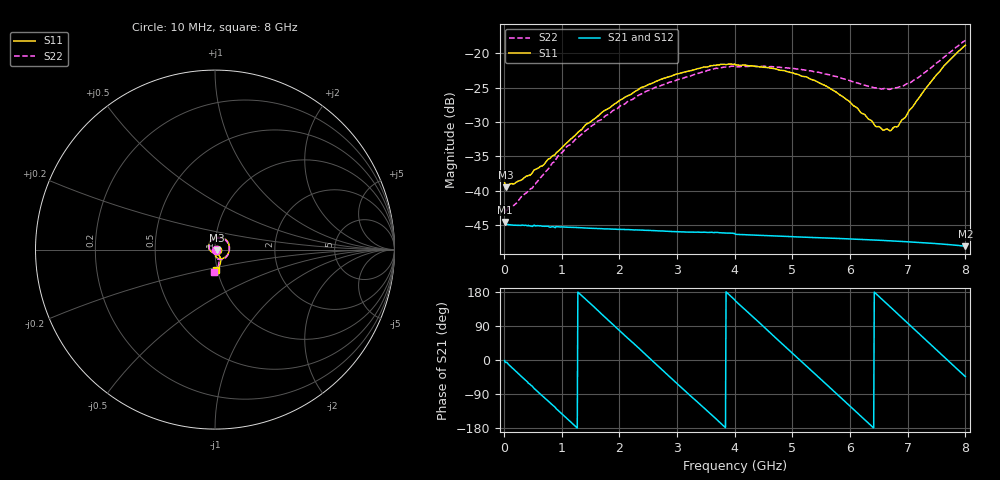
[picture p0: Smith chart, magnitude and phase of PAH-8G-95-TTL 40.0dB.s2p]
! MTS Systemtechnik GmbH
! S-Parameters
! Model: PAH-8G/95-TTL
! Attenuation Step: 40.0dB
! Rohde & Schwarz ZVB8 2Ports - Version 4.11 - 1145.1010k08 SN: 100119
! S2P File Measurements:
! S11 S21 S12 S22
# HZ  S  DB  R  50.00
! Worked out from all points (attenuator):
!   800 points, 10 MHz to 8 GHz, reference 50 ohm
!   highest |S21| = -44.56 dB at 10 MHz (marker M1); lowest = -48.1 dB at 8 GHz (marker M2)
!   lowest |S11| = -39.5 dB at 30 MHz (marker M3), VSWR 1.02, Z = 51.1 - j0.174 ohm
!   |S11| at or under -10 dB: start of sweep to end of sweep
!   |S22| runs from -43.3 to -18.1 dB; largest |S21 - S12| = 8.6e-05
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1e7  -38.85 -11.4  -44.56 -1.2  -44.46 -1.1  -42.43 -16.6
3e7  -39.54 -9.3  -44.97 -6.4  -44.99 -6.4  -43.26 -12.4
1.9e8  -38.94 -28.7  -45.04 -27.6  -45.04 -27.5  -42.01 -34.6
4.5e8  -37.79 -65.9  -45.16 -64.1  -45.17 -63.9  -39.81 -73.9
9.6e8  -34.11 -130.1  -45.29 -135.9  -45.29 -136.1  -34.76 -135.6
1.35e9  -31.06 -169.3  -45.42 169.3  -45.44 169.2  -31.75 -169.4
1.71e9  -28.52 162.2  -45.57 118.7  -45.59 119.1  -29.51 163.7
2.01e9  -26.83 140.2  -45.64 76.4  -45.67 76.6  -27.69 142.7
2.38e9  -24.97 116.1  -45.74 25.0  -45.75 25.0  -25.92 120.3
2.68e9  -23.92 97.5  -45.87 -17.3  -45.85 -17.0  -24.83 102.8
3.44e9  -22.07 53.6  -46.07 -122.6  -46.07 -123.1  -22.72 59.9
4.01e9  -21.68 20.5  -46.36 156.4  -46.37 156.3  -21.97 28.4
4.69e9  -22.24 -17.2  -46.61 61.3  -46.63 61.2  -21.99 -6.8
5.34e9  -23.83 -51.8  -46.83 -29.4  -46.85 -29.3  -22.61 -38.0
5.6e9  -24.83 -64.1  -46.92 -65.7  -46.94 -65.8  -23.05 -49.1
5.9e9  -26.47 -76.8  -47.01 -107.9  -47.03 -107.9  -23.74 -60.0
6.45e9  -30.67 -82.8  -47.21 174.9  -47.23 174.8  -25.02 -71.7
6.67e9  -31.19 -71.4  -47.29 143.8  -47.31 143.8  -25.25 -71.8
6.83e9  -30.62 -63.2  -47.37 121.3  -47.39 121.1  -24.95 -71.9
7.07e9  -27.94 -54.7  -47.49 87.3  -47.51 87.3  -24.14 -71.5
7.62e9  -21.91 -67.7  -47.81 9.7  -47.82 9.7  -20.63 -78.9
8e9  -18.83 -86.1  -48.10 -43.8  -48.12 -43.8  -18.13 -92.2
